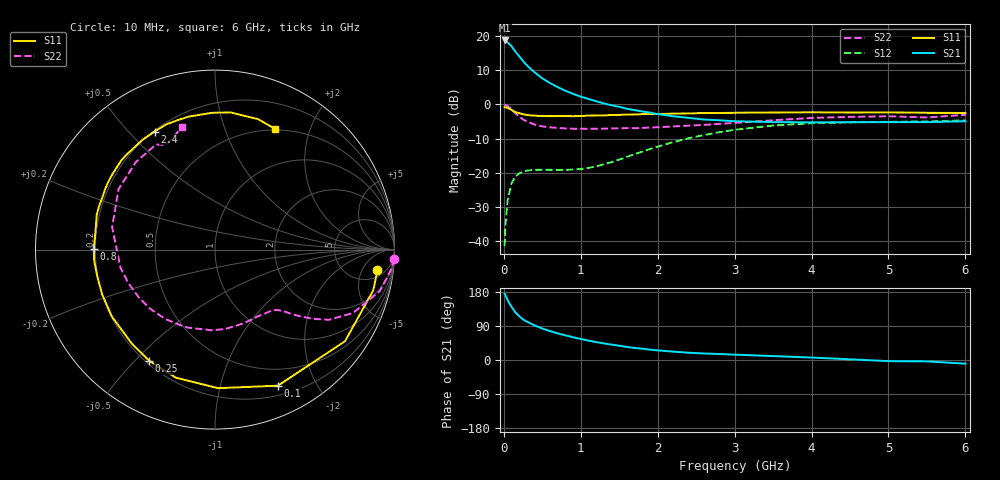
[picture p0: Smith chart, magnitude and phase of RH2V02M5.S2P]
! SIEMENS Small Signal Semiconductors
! BFR106
! Si NPN RF Bipolar Junction Transistor in SOT23
! VCE = 2 V  IC = 2.5 mA
! Common Emitter S-Parameters:  August  1996
# GHz  S  MA  R  50
!  f  S11  S21  S12  S22
! GHz  MAG  ANG  MAG  ANG  MAG  ANG  MAG  ANG
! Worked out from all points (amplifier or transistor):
!   36 points, 10 MHz to 6 GHz, reference 50 ohm
!   highest |S21| = 18.8 dB at 10 MHz (marker M1)
!   |S21| within 3 dB of that: start of sweep to 140.9 MHz
!   unconditionally stable (mu >= 1): 742.9 MHz to 2.194 GHz; 3.477 GHz to end of sweep
!   at 250 MHz: K = 0.36, MSG = 16.2 dB, |S12| = -19.7 dB
!   at 1.4 GHz: K = 1.27, MAG = 5.2 dB, |S12| = -16.9 dB
!   at 6 GHz: K = 1.02, MAG = -1.1 dB, |S12| = -4.7 dB
!   S11 on the Smith chart (normalised r, x): 10 MHz: 7, -10; 100 MHz: 0.30, -1.52; 250 MHz: 0.21, -0.55; 800 MHz: 0.19, +0.00; 2.4 GHz: 0.20, +0.59; 6 GHz: 0.49, +1.51
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0.01  0.9125 -7.3  8.718 174.7  0.0083 86.3  0.9967 -2.9
0.02  0.9104 -14.4  8.612 171.1  0.0166 81.3  0.9905 -6.0
0.05  0.8862 -35.2  8.162 157.5  0.0399 70.4  0.9472 -14.1
0.1  0.8352 -65.2  7.142 140.2  0.0699 56.0  0.8459 -24.7
0.15  0.7723 -88.7  5.975 125.5  0.0876 44.9  0.7445 -31.7
0.2  0.7461 -107.0  5.101 115.6  0.0972 38.3  0.6655 -35.4
0.25  0.7195 -120.6  4.335 107.0  0.1035 33.1  0.6022 -38.1
0.3  0.7002 -131.2  3.748 101.1  0.1069 30.4  0.5633 -39.8
0.4  0.6851 -147.0  2.96 91.2  0.1097 26.6  0.508 -42.2
0.5  0.6765 -158.3  2.422 83.0  0.11 25.5  0.4767 -44.8
0.6  0.6727 -167.2  2.061 76.2  0.1099 26.1  0.4615 -47.9
0.8  0.676 179.6  1.588 65.0  0.1096 30.6  0.445 -55.2
1.1  0.6873 163.4  1.205 51.1  0.1171 42.9  0.4401 -68.3
1.6  0.7096 143.6  0.864 34.4  0.1701 58.6  0.4499 -93.0
2.2  0.7332 123.5  0.672 22.1  0.2795 57.9  0.476 -125.7
2.4  0.7391 117.1  0.636 19.2  0.3191 54.9  0.489 -137.6
3  0.7554 101.2  0.568 14.1  0.4252 42.7  0.5364 -169.2
3.5  0.7622 91.3  0.551 10.3  0.4909 31.7  0.5863 167.7
4.5  0.7626 77.6  0.549 1.8  0.5477 12.1  0.6577 132.1
5  0.7657 71.8  0.551 -3.0  0.5563 4.7  0.6714 119.4
5.5  0.7551 67.0  0.55 -3.7  0.563 1.2  0.6446 115.1
6  0.7515 63.4  0.568 -9.6  0.5849 -6.2  0.706 105.0
